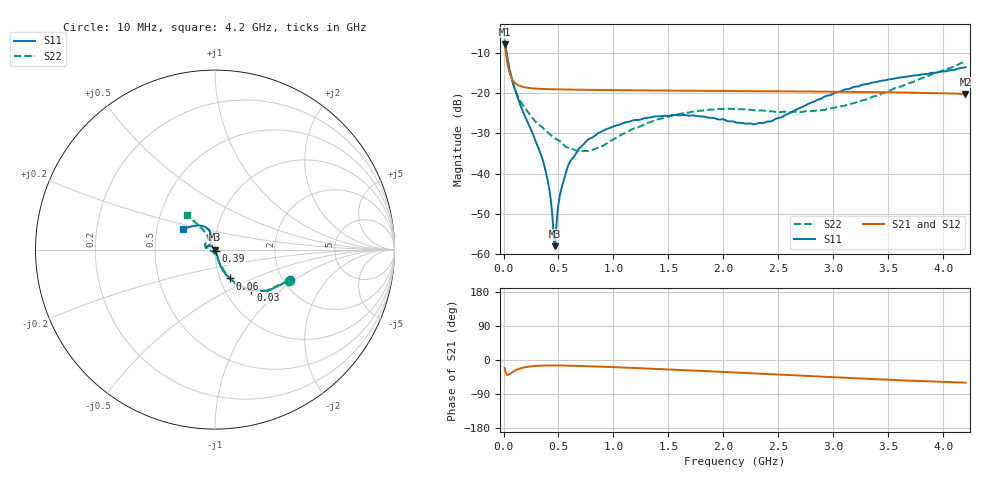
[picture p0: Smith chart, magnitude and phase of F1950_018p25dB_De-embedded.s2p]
! Integrated Device Technology
! Corporate Headquarters
! 6024 Silver Creek Valley Road
! San Jose, CA 95138  USA
! Phone:  1-408-284-8200
! Toll Free:  1-800-223-1366
! Webpage:  http://www.idt.com/
! Timing and RF Division
! 515 Groton Road, Suite 102
! Westford, MA 01886-6024
! Device:  F1950
! Description: 7-bit 0.25 dB Digital Step Attenuator
! Frequency:  150.0 -  4000.00 MHz
! Package:  4x4 mm Thin QFN Plastic Package: 24 pin
! Ports:  2 RF, 12 DC
!  Pin  1  = D0
!  Pin  2  = VDD
!  Pin  3  = Vmode
!  Pin  4  = GND
!  Pin  5  = RF1  =  Port 1
!  Pin  6  = GND
!  Pin  7  = GND
!  Pin  8  = GND
!  Pin  9  = GND
!  Pin 10  = GND
!  Pin 11  = GND
!  Pin 12  = GND
!  Pin 13  = GND
!  Pin 14  = RF2  =  Port 2
!  Pin 15  = GND
!  Pin 16  = LE
!  Pin 17  = CLK
!  Pin 18  = DATE
!  Pin 19  = D6
!  Pin 20  = D5
!  Pin 21  = D4
!  Pin 22  = D3
!  Pin 23  = D2
!  Pin 24  = D1
! State:  73
! Atten State:  18.25 dB
! Voltage:  +5.00 Volts
! Current:  Not Measured mA
! Data:  The device was measured on a the F195X evaluation board which has
!  individual transmission lines to the RF pins.  Data was collected
!  using a calibrated network analyzer.  The evaluation board was
!  de-embedded using a TRL calibration technique.
!  The reference plane is the edge of the package pin.
! Misc:  Board 2019
!  Action Tracker AT0250
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# GHz S dB R 50
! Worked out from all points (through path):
!   420 points, 10 MHz to 4.2 GHz, reference 50 ohm
!   highest |S21| = -7.76 dB at 10 MHz (marker M1); lowest = -20.2 dB at 4.2 GHz (marker M2)
!   group delay of S21, straight-line fit = 31.4 ps
!   lowest |S11| = -58.1 dB at 470 MHz (marker M3), VSWR 1.00, Z = 49.9 - j0.0108 ohm
!   |S11| at or under -10 dB: 27.73 MHz to end of sweep
!   |S22| runs from -34.5 to -7.0 dB; largest |S21 - S12| = 0.00018
!   S11 on the Smith chart (normalised r, x): 10 MHz: 2.17, -0.93; 30 MHz: 1.31, -0.65; 60 MHz: 1.12, -0.37; 390 MHz: 1.01, -0.02; 4.2 GHz: 0.68, +0.17
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0.01  -6.88 -22.1  -7.76 -21.2  -7.76 -21.2  -7.00 -22.7
0.03  -10.41 -48.5  -11.59 -38.3  -11.59 -38.3  -10.46 -48.7
0.06  -14.87 -62.8  -15.35 -36.7  -15.35 -36.7  -14.67 -62.6
0.11  -19.56 -70.5  -17.58 -27.2  -17.58 -27.2  -19.46 -68.4
0.16  -23.43 -71.7  -18.30 -21.5  -18.30 -21.5  -22.29 -72.1
0.33  -34.51 -69.8  -18.92 -15.1  -18.92 -15.1  -28.02 -78.5
0.39  -40.22 -69.0  -18.98 -14.6  -18.98 -14.6  -29.41 -80.1
0.42  -44.52 -75.4  -19.01 -14.5  -19.01 -14.5  -30.18 -81.6
0.45  -52.62 -92.6  -19.03 -14.5  -19.03 -14.5  -30.91 -85.3
0.47  -58.07 -175.0  -19.04 -14.5  -19.04 -14.5  -31.25 -88.1
0.48  -53.33 154.8  -19.05 -14.5  -19.05 -14.5  -31.40 -89.1
0.52  -44.46 138.8  -19.07 -14.6  -19.07 -14.6  -32.12 -91.7
0.57  -39.56 134.0  -19.09 -14.8  -19.09 -14.8  -33.39 -99.0
0.71  -33.19 137.5  -19.15 -15.8  -19.14 -15.9  -34.43 -123.7
0.99  -28.39 147.3  -19.24 -18.7  -19.24 -18.7  -31.65 -168.6
1.41  -25.77 163.4  -19.34 -23.8  -19.34 -23.8  -26.47 168.0
1.73  -25.55 169.1  -19.40 -27.9  -19.40 -27.9  -24.52 159.1
2.11  -27.24 158.9  -19.47 -33.1  -19.47 -33.1  -23.98 149.9
2.43  -27.02 126.7  -19.53 -37.3  -19.53 -37.3  -24.50 140.5
2.81  -22.25 105.2  -19.60 -42.7  -19.59 -42.7  -24.47 125.9
3.51  -16.55 117.6  -19.78 -52.2  -19.78 -52.2  -19.44 119.4
4.2  -13.52 146.3  -20.18 -59.7  -20.18 -59.8  -12.10 129.5
